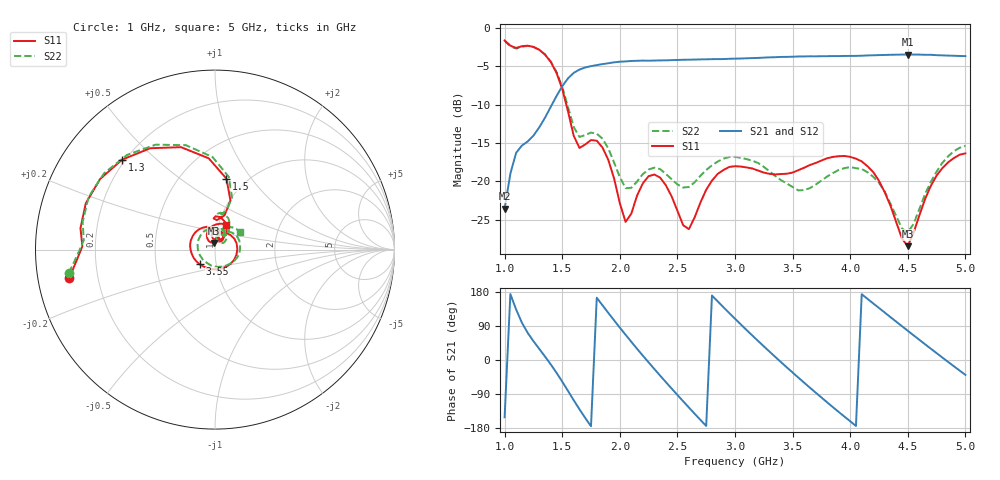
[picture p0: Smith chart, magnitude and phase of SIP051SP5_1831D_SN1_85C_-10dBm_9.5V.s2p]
# GHz  S  dB  R  50
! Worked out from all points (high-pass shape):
!   81 points, 1 GHz to 5 GHz, reference 50 ohm
!   highest |S21| = -3.48 dB at 4.5 GHz (marker M1); lowest = -23.6 dB at 1 GHz (marker M2)
!   |S21| within 3 dB of the highest: 1.558 GHz to end of sweep
!   lowest |S11| = -28.5 dB at 4.5 GHz (marker M3), VSWR 1.08, Z = 49.1 + j3.62 ohm
!   |S11| at or under -10 dB: 1.535 GHz to end of sweep
!   |S22| runs from -26.6 to -1.7 dB; largest |S21 - S12| = 0.0027
!   S11 on the Smith chart (normalised r, x): 1 GHz: 0.10, -0.10; 1.3 GHz: 0.19, +0.39; 1.5 GHz: 0.81, +0.77; 3.55 GHz: 0.83, -0.14; 5 GHz: 1.08, +0.31
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1  -1.64 -168.9  -23.60 -151.2  -23.58 -151.1  -1.68 -170.9
1.1  -2.63 178.6  -16.30 133.3  -16.25 133.2  -2.70 175.9
1.3  -2.85 135.9  -13.00 29.7  -12.99 29.7  -2.86 132.8
1.5  -7.95 80.8  -7.62 -57.0  -7.60 -57.0  -7.70 79.2
1.6  -14.08 74.5  -5.87 -106.1  -5.86 -106.1  -12.93 73.5
1.7  -15.21 92.6  -5.16 -153.0  -5.16 -153.0  -13.98 85.7
1.85  -15.61 70.8  -4.73 144.2  -4.72 144.2  -14.46 66.7
2  -22.86 57.2  -4.42 85.6  -4.40 85.6  -19.46 56.6
2.2  -20.28 98.9  -4.27 11.5  -4.27 11.6  -19.07 78.3
2.35  -19.53 69.7  -4.25 -41.2  -4.24 -41.1  -18.42 62.1
2.5  -23.85 51.2  -4.19 -92.3  -4.17 -92.2  -20.42 53.7
2.7  -22.79 82.1  -4.11 -158.1  -4.10 -158.1  -19.30 60.3
2.85  -19.05 55.5  -4.08 154.6  -4.08 154.6  -17.44 44.5
3  -18.04 15.9  -4.02 108.9  -4.00 108.9  -16.82 19.6
3.3  -19.04 -72.1  -3.85 22.0  -3.85 22.0  -18.72 -42.0
3.55  -18.56 -136.2  -3.73 -46.5  -3.74 -46.6  -21.21 -120.8
3.7  -17.63 -169.2  -3.71 -86.0  -3.70 -86.0  -20.45 -177.9
4.05  -17.06 119.2  -3.66 -174.1  -3.63 -174.2  -18.31 85.8
4.35  -23.22 71.8  -3.51 113.1  -3.52 113.2  -22.97 38.8
4.5  -28.48 102.3  -3.48 77.1  -3.48 77.2  -26.65 62.9
4.75  -19.27 112.8  -3.56 18.2  -3.55 18.1  -18.76 74.0
5  -16.37 67.0  -3.68 -39.2  -3.68 -39.2  -15.39 35.8
